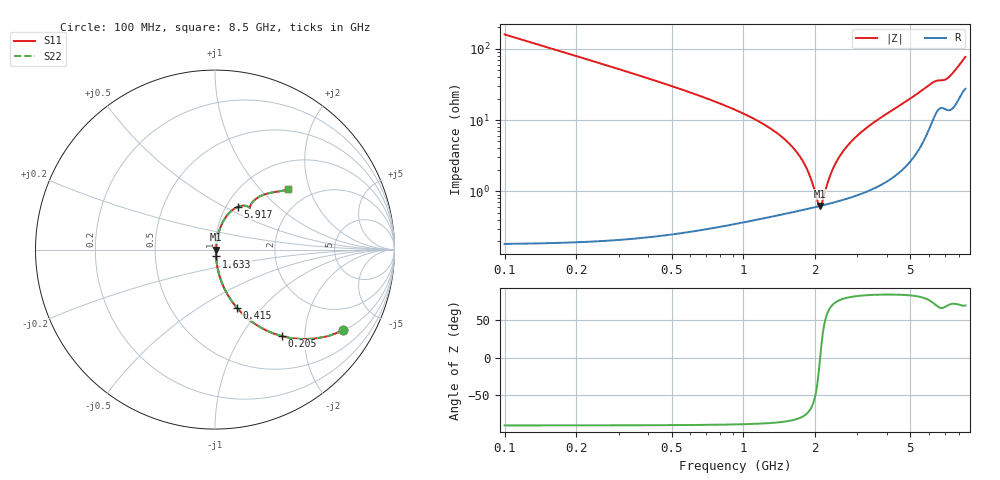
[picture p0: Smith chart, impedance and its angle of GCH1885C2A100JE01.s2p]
!Murata Part Number: GCH1885C2A100JE01
!These Parameters are Measured in Series Mode Connection
!Data Generated on Mar 13, 2026
!  o--ll--o
!Port1  Port2
!  o------o
!Operation Temp=25[degC], DC Bias Voltage=0[V]
!Freq. Start=100[MHz] Stop=9[GHz] 401[Steps]
# Hz S RI R 50
!Freq.(Hz) S11(Real) S11(Imag) S21(Real) S21(Imag) S12(Real) S12(Imag) S22(Real) S22(Imag)
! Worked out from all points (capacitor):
!   401 points, 100 MHz to 8.5 GHz, reference 50 ohm
!   read as one part in series: C = 10 pF near 142 MHz
!   lowest |Z| = 622 mohm at 2.095 GHz (marker M1)
!   series resonance near 2.095 GHz, so ESL is about 580 pH
!   S11 on the Smith chart (normalised r, x): 100 MHz: 1.00, -3.18; 205 MHz: 1.00, -1.54; 415 MHz: 1.00, -0.74; 1.633 GHz: 1.01, -0.08; 5.917 GHz: 1.14, +0.59; 8.5 GHz: 1.55, +1.44
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1e8  0.7158 -0.4505  0.2842 0.4505  0.2842 0.4505  0.7158 -0.4505
2.05e8  0.3718 -0.482  0.6282 0.482  0.6282 0.482  0.3718 -0.482
2.89e8  0.2266 -0.4168  0.7734 0.4168  0.7734 0.4168  0.2266 -0.4168
4.15e8  0.1209 -0.3229  0.8791 0.3229  0.8791 0.3229  0.1209 -0.3229
8.14e8  0.0297 -0.1605  0.9702 0.1605  0.9702 0.1605  0.0297 -0.1605
1.507e9  0.00743 -0.0508  0.9926 0.0508  0.9926 0.0508  0.00743 -0.0508
1.633e9  0.00659 -0.0383  0.9934 0.0383  0.9934 0.0383  0.00659 -0.0383
1.843e9  0.00598 -0.0197  0.994 0.0197  0.994 0.0197  0.00598 -0.0197
2.053e9  0.00609 -0.00314  0.9939 0.00314  0.9939 0.00314  0.00609 -0.00314
2.095e9  0.00618 -2.75e-05  0.9938 2.75e-05  0.9938 2.75e-05  0.00618 -2.75e-05
2.137e9  0.00629 0.00303  0.9937 -0.00303  0.9937 -0.00303  0.00629 0.00303
2.305e9  0.00692 0.0148  0.9931 -0.0148  0.9931 -0.0148  0.00692 0.0148
2.431e9  0.00756 0.0233  0.9924 -0.0233  0.9924 -0.0233  0.00756 0.0233
2.641e9  0.00895 0.0367  0.991 -0.0367  0.991 -0.0367  0.00895 0.0367
2.914e9  0.0113 0.0535  0.9887 -0.0535  0.9887 -0.0535  0.0113 0.0535
3.481e9  0.0183 0.0871  0.9817 -0.0871  0.9817 -0.0871  0.0183 0.0871
4.3e9  0.0353 0.1363  0.9647 -0.1363  0.9647 -0.1363  0.0353 0.1363
5.707e9  0.1081 0.2284  0.8919 -0.2284  0.8919 -0.2284  0.1081 0.2284
5.917e9  0.1289 0.239  0.8711 -0.239  0.8711 -0.239  0.1289 0.239
6.505e9  0.1884 0.2367  0.8116 -0.2367  0.8116 -0.2367  0.1884 0.2367
7.114e9  0.1993 0.2494  0.8007 -0.2494  0.8007 -0.2494  0.1993 0.2494
8.5e9  0.4047 0.3356  0.5953 -0.3356  0.5953 -0.3356  0.4047 0.3356
